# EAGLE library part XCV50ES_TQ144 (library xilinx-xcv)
xcv50es_tq144 edit this description Auto generated by make-symbol-device-package-bsdl.ulp Rev. 26 Source: xcv50es_tq144.bsd
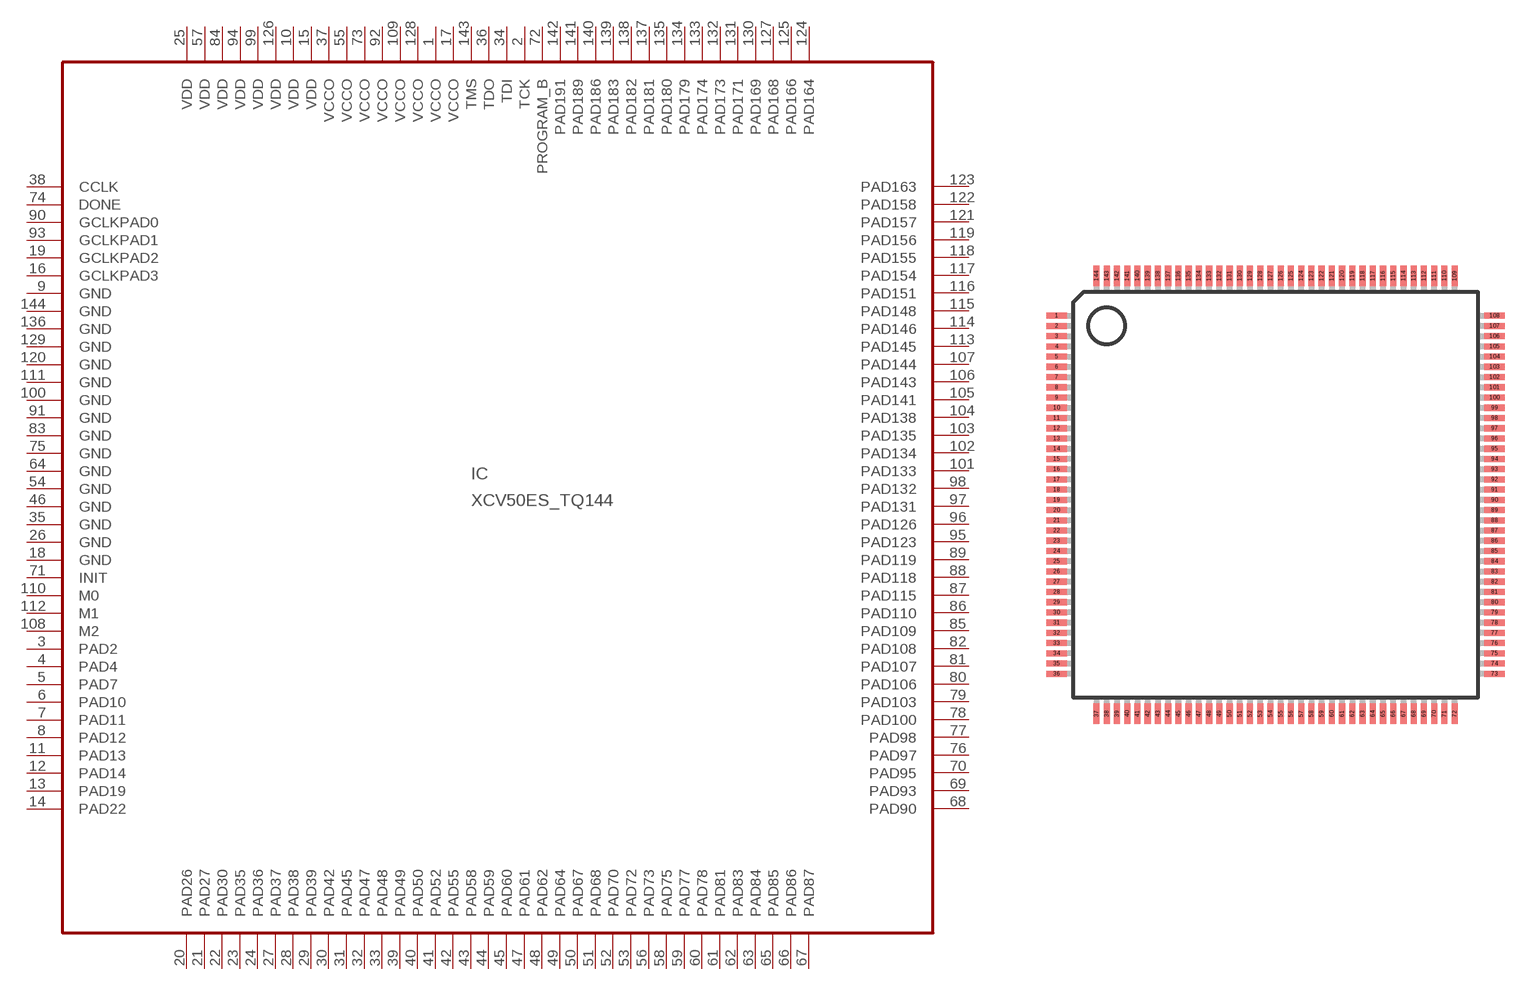
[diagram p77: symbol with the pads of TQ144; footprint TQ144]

Designator prefix IC

## XCV50ES_TQ144 (OC_FARNELL: unknown; OC_NEWARK: unknown)  [TQ144]
1  VCCO  pwr
2  TCK  in
3  PAD2
4  PAD4
5  PAD7
6  PAD10
7  PAD11
8  PAD12
9  GND  pwr
10  VDD  pwr
11  PAD13
12  PAD14
13  PAD19
14  PAD22
15  VDD  pwr
16  GCLKPAD3  in
17  VCCO  pwr
18  GND  pwr
19  GCLKPAD2  in
20  PAD26
21  PAD27
22  PAD30
23  PAD35
24  PAD36
25  VDD  pwr
26  GND  pwr
27  PAD37
28  PAD38
29  PAD39
30  PAD42
31  PAD45
32  PAD47
33  PAD48
34  TDI  in
35  GND  pwr
36  TDO  out
37  VCCO  pwr
38  CCLK
39  PAD49
40  PAD50
41  PAD52
42  PAD55
43  PAD58
44  PAD59
45  PAD60
46  GND  pwr
47  PAD61
48  PAD62
49  PAD64
50  PAD67
51  PAD68
52  PAD70
53  PAD72
54  GND  pwr
55  VCCO  pwr
56  PAD73
57  VDD  pwr
58  PAD75
59  PAD77
60  PAD78
61  PAD81
62  PAD83
63  PAD84
64  GND  pwr
65  PAD85
66  PAD86
67  PAD87
68  PAD90
69  PAD93
70  PAD95
71  INIT
72  PROGRAM_B  in
73  VCCO  pwr
74  DONE
75  GND  pwr
76  PAD97
77  PAD98
78  PAD100
79  PAD103
80  PAD106
81  PAD107
82  PAD108
83  GND  pwr
84  VDD  pwr
85  PAD109
86  PAD110
87  PAD115
88  PAD118
89  PAD119
90  GCLKPAD0  in
91  GND  pwr
92  VCCO  pwr
93  GCLKPAD1  in
94  VDD  pwr
95  PAD123
96  PAD126
97  PAD131
98  PAD132
99  VDD  pwr
100  GND  pwr
101  PAD133
102  PAD134
103  PAD135
104  PAD138
105  PAD141
106  PAD143
107  PAD144
108  M2  in
109  VCCO  pwr
110  M0  in
111  GND  pwr
112  M1  in
113  PAD145
114  PAD146
115  PAD148
116  PAD151
117  PAD154
118  PAD155
119  PAD156
120  GND  pwr
121  PAD157
122  PAD158
123  PAD163
124  PAD164
125  PAD166
126  VDD  pwr
127  PAD168
128  VCCO  pwr
129  GND  pwr
130  PAD169
131  PAD171
132  PAD173
133  PAD174
134  PAD179
135  PAD180
136  GND  pwr
137  PAD181
138  PAD182
139  PAD183
140  PAD186
141  PAD189
142  PAD191
143  TMS  in
144  GND  pwr

## Footprint TQ144 (pad centres in mm)
TQ144 Auto generated by make-symbol-device-package-bsdl.ulp Rev. 26 Source: xcv100_tq144_1532.bsd; tq144.pdf
smd 1 x 0.3: 1 -10.7,8.75; 2 -10.7,8.25; 3 -10.7,7.75; 4 -10.7,7.25; 5 -10.7,6.75; 6 -10.7,6.25; 7 -10.7,5.75; 8 -10.7,5.25; 9 -10.7,4.75; 10 -10.7,4.25; 11 -10.7,3.75; 12 -10.7,3.25; 13 -10.7,2.75; 14 -10.7,2.25; 15 -10.7,1.75; 16 -10.7,1.25; 17 -10.7,0.75; 18 -10.7,0.25; 19 -10.7,-0.25; 20 -10.7,-0.75; 21 -10.7,-1.25; 22 -10.7,-1.75; 23 -10.7,-2.25; 24 -10.7,-2.75; 25 -10.7,-3.25; 26 -10.7,-3.75; 27 -10.7,-4.25; 28 -10.7,-4.75; 29 -10.7,-5.25; 30 -10.7,-5.75; 31 -10.7,-6.25; 32 -10.7,-6.75; 33 -10.7,-7.25; 34 -10.7,-7.75; 35 -10.7,-8.25; 36 -10.7,-8.75; 73 10.7,-8.75; 74 10.7,-8.25; 75 10.7,-7.75; 76 10.7,-7.25; 77 10.7,-6.75; 78 10.7,-6.25; 79 10.7,-5.75; 80 10.7,-5.25; 81 10.7,-4.75; 82 10.7,-4.25; 83 10.7,-3.75; 84 10.7,-3.25; 85 10.7,-2.75; 86 10.7,-2.25; 87 10.7,-1.75; 88 10.7,-1.25; 89 10.7,-0.75; 90 10.7,-0.25; 91 10.7,0.25; 92 10.7,0.75; 93 10.7,1.25; 94 10.7,1.75; 95 10.7,2.25; 96 10.7,2.75; 97 10.7,3.25; 98 10.7,3.75; 99 10.7,4.25; 100 10.7,4.75; 101 10.7,5.25; 102 10.7,5.75; 103 10.7,6.25; 104 10.7,6.75; 105 10.7,7.25; 106 10.7,7.75; 107 10.7,8.25; 108 10.7,8.75
smd 0.3 x 1: 37 -8.75,-10.7; 38 -8.25,-10.7; 39 -7.75,-10.7; 40 -7.25,-10.7; 41 -6.75,-10.7; 42 -6.25,-10.7; 43 -5.75,-10.7; 44 -5.25,-10.7; 45 -4.75,-10.7; 46 -4.25,-10.7; 47 -3.75,-10.7; 48 -3.25,-10.7; 49 -2.75,-10.7; 50 -2.25,-10.7; 51 -1.75,-10.7; 52 -1.25,-10.7; 53 -0.75,-10.7; 54 -0.25,-10.7; 55 0.25,-10.7; 56 0.75,-10.7; 57 1.25,-10.7; 58 1.75,-10.7; 59 2.25,-10.7; 60 2.75,-10.7; 61 3.25,-10.7; 62 3.75,-10.7; 63 4.25,-10.7; 64 4.75,-10.7; 65 5.25,-10.7; 66 5.75,-10.7; 67 6.25,-10.7; 68 6.75,-10.7; 69 7.25,-10.7; 70 7.75,-10.7; 71 8.25,-10.7; 72 8.75,-10.7; 109 8.75,10.7; 110 8.25,10.7; 111 7.75,10.7; 112 7.25,10.7; 113 6.75,10.7; 114 6.25,10.7; 115 5.75,10.7; 116 5.25,10.7; 117 4.75,10.7; 118 4.25,10.7; 119 3.75,10.7; 120 3.25,10.7; 121 2.75,10.7; 122 2.25,10.7; 123 1.75,10.7; 124 1.25,10.7; 125 0.75,10.7; 126 0.25,10.7; 127 -0.25,10.7; 128 -0.75,10.7; 129 -1.25,10.7; 130 -1.75,10.7; 131 -2.25,10.7; 132 -2.75,10.7; 133 -3.25,10.7; 134 -3.75,10.7; 135 -4.25,10.7; 136 -4.75,10.7; 137 -5.25,10.7; 138 -5.75,10.7; 139 -6.25,10.7; 140 -6.75,10.7; 141 -7.25,10.7; 142 -7.75,10.7; 143 -8.25,10.7; 144 -8.75,10.7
